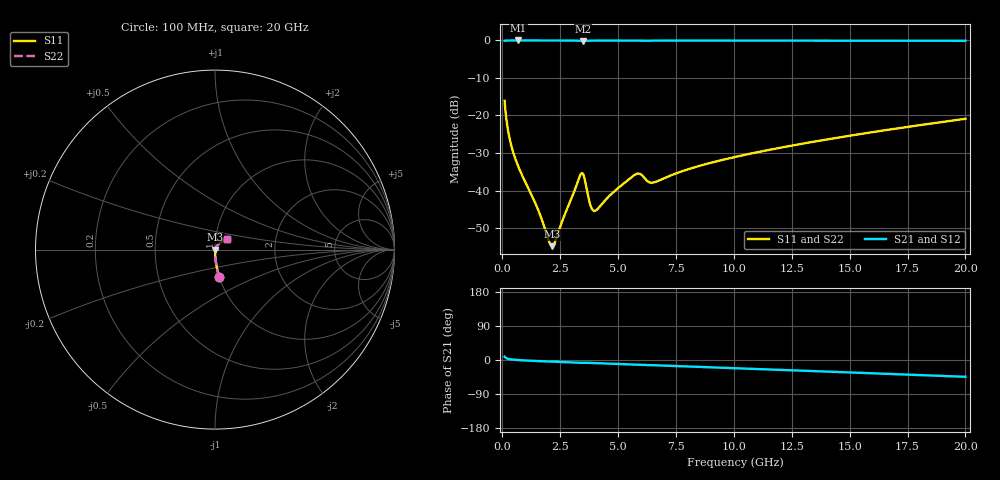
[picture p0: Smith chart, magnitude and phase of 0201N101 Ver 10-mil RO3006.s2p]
# GHz S MA R 50
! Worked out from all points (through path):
!   1601 points, 100 MHz to 20 GHz, reference 50 ohm
!   highest |S21| = -0.01 dB at 697 MHz (marker M1); lowest = -0.1 dB at 3.483 GHz (marker M2)
!   group delay of S21, straight-line fit = 6.27 ps
!   lowest |S11| = -54.8 dB at 2.152 GHz (marker M3), VSWR 1.00, Z = 50.2 - j0.031 ohm
!   |S11| at or under -10 dB: start of sweep to end of sweep
!   |S22| runs from -54.8 to -16.1 dB; largest |S21 - S12| = 0
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0.1  0.1565 -81.0  0.9872 8.8  0.9872 8.8  0.1565 -81.0
0.34875  0.04442 -87.4  0.9984 1.8  0.9984 1.8  0.04442 -87.4
0.697  0.02065 -87.9  0.9989 -0.2  0.9989 -0.2  0.02065 -87.9
1.530312  0.005696 -78.5  0.9985 -2.8  0.9985 -2.8  0.005696 -78.5
2.027813  0.00206 -37.6  0.9982 -4.0  0.9982 -4.0  0.00206 -37.6
2.152188  0.001812 -9.8  0.9981 -4.3  0.9981 -4.3  0.001812 -9.8
2.289  0.002099 19.8  0.998 -4.7  0.998 -4.7  0.002099 19.8
3.296438  0.01412 45.9  0.9914 -7.3  0.9914 -7.3  0.01412 45.9
3.420812  0.01699 26.1  0.9857 -7.4  0.9857 -7.4  0.01699 26.1
3.483  0.01669 12.3  0.9842 -7.3  0.9842 -7.3  0.01669 12.3
3.570063  0.01365 -4.0  0.9863 -7.2  0.9863 -7.2  0.01365 -4.0
3.806375  0.006353 -1.7  0.9936 -7.7  0.9936 -7.7  0.006353 -1.7
3.9805  0.00533 21.7  0.9953 -8.2  0.9953 -8.2  0.00533 21.7
5.759062  0.01644 50.9  0.9924 -12.4  0.9924 -12.4  0.01644 50.9
5.9705  0.0165 41.3  0.9901 -12.8  0.9901 -12.8  0.0165 41.3
6.380937  0.01279 42.9  0.9927 -13.4  0.9927 -13.4  0.01279 42.9
6.741625  0.01346 53.2  0.9946 -14.3  0.9946 -14.3  0.01346 53.2
8.10975  0.01956 60.4  0.9955 -17.4  0.9955 -17.4  0.01956 60.4
10.05  0.02796 59.3  0.995 -21.7  0.995 -21.7  0.02796 59.3
13.37081  0.04426 54.4  0.9937 -29.1  0.9937 -29.1  0.04426 54.4
16.69162  0.06465 48.3  0.9918 -36.7  0.9918 -36.7  0.06465 48.3
20  0.09024 41.6  0.989 -44.3  0.989 -44.3  0.09024 41.6
